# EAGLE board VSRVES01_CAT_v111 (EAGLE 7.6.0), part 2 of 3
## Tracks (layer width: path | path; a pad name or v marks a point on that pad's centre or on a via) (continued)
D4  (via drill 0.2) (continued)
  Top 0.11: TP_D8.TP 26.8,25.2 arc90 26.9,25.1 26.91,25.1 arc-90 27.01,25 27.01,25 arc-90 26.91,24.89 26.69,24.89 arc90 26.59,24.8 26.59,24.79 arc90 26.69,24.69 26.91,24.69 arc-90 27.01,24.59 27.01,24.59 arc-90 26.91,24.48 26.69,24.48 arc90 26.59,24.39 26.59,24.38 arc90 26.69,24.28 26.91,24.28 arc-90 27.01,24.18 27.01,24.18 arc-90 26.91,24.07 26.69,24.07 arc90 26.59,23.98 26.59,23.97 arc90 26.69,23.87 26.91,23.87 arc-90 27.01,23.77 27.01,23.77 arc-90 26.91,23.67 26.69,23.67 arc90 26.59,23.57 26.59,23.56 arc90 26.69,23.46 26.91,23.46 arc-90 27.01,23.36 27.01,23.36 arc-90 26.91,23.26 26.69,23.26 arc90 26.59,23.16 26.59,23.15 arc90 26.69,23.05 26.91,23.05 arc-90 27.01,22.95 27.01,22.95 arc-90 26.91,22.85 26.69,22.85 arc90 26.59,22.75 26.59,22.74 arc90 26.69,22.64 26.91,22.64 arc-90 27.01,22.54 27.01,22.54 arc-90 26.91,22.44 26.69,22.44 arc90 26.59,22.34 26.59,22.33 arc90 26.69,22.23 26.91,22.23 arc-90 27.01,22.13 27.01,22.13 arc-90 26.91,22.03 26.69,22.03 arc90 26.59,21.93 26.59,21.92 arc90 26.69,21.82 26.91,21.82 arc-90 27.01,21.72 27.01,21.72 arc-90 26.91,21.62 26.69,21.62 arc90 26.59,21.52 26.59,21.51 arc90 26.69,21.41 26.91,21.41 arc-90 27.01,21.31 27.01,21.31 arc-90 26.91,21.21 26.69,21.21 arc90 26.59,21.11 26.59,21.1 arc90 26.69,21 26.91,21 arc-90 27.01,20.9 27.01,20.9 arc-90 26.91,20.8 26.69,20.8 arc90 26.59,20.7 26.59,20.69 arc90 26.69,20.59 26.91,20.59 arc-90 27.01,20.49 27.01,20.49 arc-90 26.91,20.39 26.69,20.39 arc90 26.59,20.29 26.59,20.28 arc90 26.69,20.18 26.91,20.18 arc-90 27.01,20.08 27.01,20.08 arc-90 26.91,19.98 26.69,19.98 arc90 26.59,19.88 26.59,19.87 arc90 26.69,19.77 26.91,19.77 arc-90 27.01,19.67 27.01,19.67 arc-90 26.91,19.57 26.69,19.57 arc90 26.59,19.47 26.59,19.46 arc90 26.69,19.36 26.91,19.36 arc-90 27.01,19.26 27.01,19.26 arc-90 26.91,19.16 26.69,19.16 arc90 26.59,19.06 26.59,19.05 arc90 26.69,18.95 26.91,18.95 arc-90 27.01,18.85 27.01,18.85 arc-90 26.91,18.75 26.69,18.75 arc90 26.59,18.65 26.59,18.64 arc90 26.69,18.54 26.91,18.54 arc-90 27.01,18.44 27.01,18.44 arc-90 26.91,18.34 26.69,18.34 arc90 26.59,18.24 26.59,18.23 arc90 26.69,18.13 26.91,18.13 arc-90 27.01,18.03 27.01,18.03 arc-90 26.91,17.93 26.69,17.93 arc90 26.59,17.83 26.59,17.82 arc90 26.69,17.72 26.91,17.72 arc-90 27.01,17.62 27.01,17.62 arc-90 26.91,17.52 26.69,17.52 arc90 26.59,17.42 26.59,17.41 arc90 26.69,17.31 26.91,17.31 arc-90 27.01,17.21 27.01,17.21 arc-90 26.91,17.11 26.69,17.11 arc90 26.59,17.01 26.59,17 arc90 26.69,16.9 26.91,16.9 arc-90 27.01,16.8 27.01,16.8 arc-90 26.91,16.7 26.9,16.7 arc90 26.8,16.6 26.8,15.88 arc-90 v24.93,14
  Top 0.11: TP_D8.TP 26.8,26.4 TP_D8.TP | U1.26 26.4,27.76 26.4,27.2 26.8,26.8 TP_D8.TP
  Bottom 0.11: U100.M6 23.98,13.71 arc-45 24.69,14 v24.93,14
D5  (via drill 0.2)
  Top 0.11: v23.62,13.35 25.64,15.36 | 25.64,15.36 25.71,15.43 25.76,15.48 25.76,16.92 25.9,17.06 25.9,17.31 arc-90 26.1,17.47 26.13,17.47 arc90 26.23,17.57 26.23,17.57 arc90 26.13,17.68 25.87,17.68 arc-90 25.77,17.77 25.77,17.78 arc-90 25.87,17.88 26.13,17.88 arc90 26.23,17.98 26.23,17.99 arc90 26.13,18.09 25.87,18.09 arc-90 25.77,18.19 25.77,18.19 arc-90 25.87,18.29 26.13,18.29 arc90 26.23,18.39 26.23,18.4 arc90 26.13,18.5 25.87,18.5 arc-90 25.77,18.6 25.77,18.61 arc-90 25.87,18.7 26.13,18.7 arc90 26.23,18.8 26.23,18.81 arc90 26.13,18.91 25.87,18.91 arc-90 25.77,19.01 25.77,19.02 arc-90 25.87,19.12 26.13,19.12 arc90 26.23,19.22 26.23,19.22 arc90 26.13,19.32 25.87,19.32 arc-90 25.77,19.42 25.77,19.43 arc-90 25.87,19.53 26.13,19.53 arc90 26.23,19.63 26.23,19.63 arc90 26.13,19.73 25.87,19.73 arc-90 25.77,19.83 25.77,19.84 arc-90 25.87,19.94 26.13,19.94 arc90 26.23,20.04 26.23,20.05 arc90 26.13,20.15 25.87,20.15 arc-90 25.77,20.25 25.77,20.25 arc-90 25.87,20.35 26.13,20.35 arc90 26.23,20.45 26.23,20.46 arc90 26.13,20.56 25.87,20.56 arc-90 25.77,20.66 25.77,20.66 arc-90 25.87,20.76 26.13,20.76 arc90 26.23,20.86 26.23,20.87 arc90 26.13,20.97 25.87,20.97 arc-90 25.77,21.07 25.77,21.08 arc-90 25.87,21.18 26.13,21.18 arc90 26.23,21.28 26.23,21.28 arc90 26.13,21.38 25.87,21.38 arc-90 25.77,21.48 25.77,21.49 arc-90 25.87,21.59 26.13,21.59 arc90 26.23,21.69 26.23,21.69 arc90 26.13,21.79 25.87,21.79 arc-90 25.77,21.89 25.77,21.9 arc-90 25.87,22 26.13,22 arc90 26.23,22.1 26.23,22.11 arc90 26.13,22.2 25.87,22.2 arc-90 25.77,22.3 25.77,22.31 arc-90 25.87,22.41 26.13,22.41 arc90 26.23,22.51 26.23,22.52 arc90 26.13,22.62 25.87,22.62 arc-90 25.77,22.72 25.77,22.72 arc-90 25.87,22.82 26.13,22.82 arc90 26.23,22.92 26.23,22.93 arc90 26.13,23.03 25.87,23.03 arc-90 25.77,23.13 25.77,23.14 arc-90 25.87,23.23 26.13,23.23 arc90 26.23,23.34 26.23,23.34 arc90 26.13,23.44 25.87,23.44 arc-90 25.77,23.54 25.77,23.55 arc-90 25.87,23.65 26.13,23.65 arc90 26.23,23.75 26.23,23.75 arc90 26.13,23.85 25.87,23.85 arc-90 25.77,23.95 25.77,23.96 arc-90 25.87,24.06 26.13,24.06 arc90 26.23,24.16 26.23,24.16 arc90 26.13,24.27 25.87,24.27 arc-90 25.77,24.36 25.77,24.37 arc-90 25.87,24.47 26.13,24.47 arc90 26.23,24.57 26.23,24.58 arc90 26.13,24.68 25.87,24.68 arc-90 25.77,24.78 25.77,24.78 arc-90 25.87,24.88 26.13,24.88 arc90 26.23,24.98 26.23,24.99 arc90 26.13,25.09 25.87,25.09 arc-90 25.77,25.19 25.77,25.19 arc-90 25.87,25.29 26.13,25.29 arc90 26.23,25.39 26.23,25.4 arc90 26.13,25.5 26.1,25.5 arc-90 26,25.6 26,26.4 26,27.59 U1.25
  Top 0.11: TP_D15.TP 25.81,15.19 25.64,15.36
  Bottom 0.11: U100.L7 v23.62,13.35
D6  (via drill 0.2)
  Top 0.11: U1.24 25.6,27.43 25.6,27.2 25.2,26.8 25.2,26.4 | v22.8,12.37 22.98,12.44 22.98,12.94 arc-45 23.27,13.64 24.91,15.28 25.47,15.84 25.47,16.48 25.2,16.75 25.2,17.06 arc-90 25.3,17.16 25.36,17.16 arc90 25.46,17.26 25.46,17.27 arc90 25.36,17.37 25.04,17.37 arc-90 24.94,17.47 24.94,17.48 arc-90 25.04,17.58 25.36,17.58 arc90 25.46,17.68 25.46,17.69 arc90 25.36,17.79 25.04,17.79 arc-90 24.94,17.89 24.94,17.9 arc-90 25.04,18 25.36,18 arc90 25.46,18.1 25.46,18.11 arc90 25.36,18.21 25.04,18.21 arc-90 24.94,18.31 24.94,18.32 arc-90 25.04,18.42 25.36,18.42 arc90 25.46,18.52 25.46,18.53 arc90 25.36,18.63 25.04,18.63 arc-90 24.94,18.73 24.94,18.74 arc-90 25.04,18.84 25.36,18.84 arc90 25.46,18.94 25.46,18.95 arc90 25.36,19.05 25.04,19.05 arc-90 24.94,19.15 24.94,19.16 arc-90 25.04,19.26 25.36,19.26 arc90 25.46,19.36 25.46,19.37 arc90 25.36,19.47 25.04,19.47 arc-90 24.94,19.57 24.94,19.58 arc-90 25.04,19.68 25.36,19.68 arc90 25.46,19.78 25.46,19.79 arc90 25.36,19.89 25.04,19.89 arc-90 24.94,19.99 24.94,20 arc-90 25.04,20.1 25.36,20.1 arc90 25.46,20.2 25.46,20.21 arc90 25.36,20.32 25.04,20.32 arc-90 24.94,20.41 24.94,20.43 arc-90 25.04,20.52 25.36,20.52 arc90 25.46,20.62 25.46,20.64 arc90 25.36,20.73 25.04,20.73 arc-90 24.94,20.84 24.94,20.85 arc-90 25.04,20.95 25.36,20.95 arc90 25.46,21.05 25.46,21.06 arc90 25.36,21.16 25.04,21.16 arc-90 24.94,21.26 24.94,21.27 arc-90 25.04,21.37 25.36,21.37 arc90 25.46,21.47 25.46,21.48 arc90 25.36,21.58 25.04,21.58 arc-90 24.94,21.68 24.94,21.69 arc-90 25.04,21.79 25.36,21.79 arc90 25.46,21.89 25.46,21.9 arc90 25.36,22 25.04,22 arc-90 24.94,22.1 24.94,22.11 arc-90 25.04,22.21 25.36,22.21 arc90 25.46,22.31 25.46,22.32 arc90 25.36,22.42 25.04,22.42 arc-90 24.94,22.52 24.94,22.53 arc-90 25.04,22.63 25.36,22.63 arc90 25.46,22.73 25.46,22.74 arc90 25.36,22.84 25.04,22.84 arc-90 24.94,22.94 24.94,22.95 arc-90 25.04,23.05 25.36,23.05 arc90 25.46,23.15 25.46,23.16 arc90 25.36,23.26 25.04,23.26 arc-90 24.94,23.36 24.94,23.37 arc-90 25.04,23.47 25.36,23.47 arc90 25.46,23.57 25.46,23.58 25.46,23.74 25.2,24 TP_D7.TP
  Top 0.11: TP_D7.TP 25.2,26.4 | 25.2,26.4 TP_D7.TP
  Bottom 0.11: U100.L8 v22.8,12.37
D7  (via drill 0.2)
  Top 0.11: 24.4,15.61 24.51,16.05 arc90 24.41,16.15 arc-90 24.31,16.25 24.31,16.27 arc-90 24.41,16.37 24.61,16.37 arc90 24.71,16.47 24.71,16.49 arc90 24.61,16.59 24.41,16.59 arc-90 24.31,16.69 24.31,16.7 arc-90 24.41,16.8 24.61,16.8 arc90 24.71,16.91 24.71,16.92 arc90 24.61,17.02 24.41,17.02 arc-90 24.31,17.12 24.31,17.14 arc-90 24.41,17.24 24.61,17.24 arc90 24.71,17.34 24.71,17.36 arc90 24.61,17.46 24.41,17.46 arc-90 24.31,17.56 24.31,17.58 arc-90 24.41,17.68 24.61,17.68 arc90 24.71,17.78 24.71,17.8 arc90 24.61,17.9 24.41,17.9 arc-90 24.31,18 24.31,18.01 arc-90 24.41,18.11 24.61,18.11 arc90 24.71,18.21 24.71,18.23 arc90 24.61,18.33 24.41,18.33 arc-90 24.31,18.43 24.31,18.45 arc-90 24.41,18.55 24.61,18.55 arc90 24.71,18.65 24.71,18.67 arc90 24.61,18.77 24.41,18.77 arc-90 24.31,18.87 24.31,18.89 arc-90 24.41,18.99 24.61,18.99 arc90 24.71,19.09 24.71,19.1 arc90 24.61,19.2 24.41,19.2 arc-90 24.31,19.3 24.31,19.32 arc-90 24.41,19.42 24.61,19.42 arc90 24.71,19.52 24.71,19.54 arc90 24.61,19.64 24.41,19.64 arc-90 24.31,19.74 24.31,19.76 arc-90 24.41,19.86 24.61,19.86 arc90 24.71,19.96 24.71,19.98 arc90 24.61,20.08 24.41,20.08 arc-90 24.31,20.18 24.31,20.2 arc-90 24.41,20.3 24.61,20.3 arc90 24.71,20.39 24.71,20.41 arc90 24.61,20.51 24.41,20.51 arc-90 24.31,20.61 24.31,20.63 arc-90 24.41,20.73 24.61,20.73 arc90 24.71,20.83 24.71,20.85 arc90 24.61,20.95 24.41,20.95 arc-90 24.31,21.05 24.31,21.07 arc-90 24.41,21.17 24.61,21.17 arc90 24.71,21.27 24.71,21.29 arc90 24.61,21.39 24.41,21.39 arc-90 24.31,21.49 24.31,21.5 arc-90 24.41,21.6 24.61,21.6 arc90 24.71,21.7 24.71,21.72 arc90 24.61,21.82 24.41,21.82 arc-90 24.31,21.92 24.31,21.94 arc-90 24.41,22.04 24.61,22.04 arc90 24.71,22.14 24.71,22.16 arc90 24.61,22.26 24.41,22.26 arc-90 24.31,22.36 24.31,22.38 arc-90 24.41,22.48 24.61,22.48 arc90 24.71,22.58 24.71,22.59 arc90 24.61,22.69 24.41,22.69 arc-90 24.31,22.79 24.31,22.81 arc-90 24.41,22.91 24.61,22.91 arc90 24.71,23.01 24.71,23.03 arc90 24.61,23.13 24.41,23.13 arc-90 24.31,23.23 24.31,23.25 arc-90 24.41,23.35 24.61,23.35 arc90 24.71,23.45 24.71,23.47 arc90 24.61,23.57 24.41,23.57 arc-90 24.31,23.67 24.31,23.68 arc-90 24.41,23.79 24.61,23.79 arc90 24.71,23.89 24.71,23.9 arc90 24.61,24 24.41,24 arc-90 24.31,24.1 24.31,24.12 arc-90 24.41,24.22 24.61,24.22 arc90 24.71,24.32 24.71,24.34 arc90 24.61,24.44 24.41,24.44 arc-90 24.31,24.54 24.31,24.56 arc-90 24.41,24.66 24.61,24.66 arc90 24.71,24.76 24.71,24.78 arc90 24.61,24.88 24.41,24.88 arc-90 24.31,24.98 24.31,24.99 arc-90 24.41,25.09 24.61,25.09 arc90 24.71,25.19 24.71,25.21 arc90 24.61,25.31 24.41,25.31 arc-90 24.31,25.41 24.31,25.43 arc-90 24.41,25.53 arc90 24.51,25.63 24.51,26.26 24.4,26.37 24.4,27 24.89,27.5 U1.23
  Top 0.11: 24.4,15.61 arc-45 24.11,14.91 22.79,13.59 arc103 v22.57,13.11 | TP_D14.TP 24.34,15.55 24.4,15.61
  Bottom 0.11: 23.27,11.72 U100.L9 23.23,11.8 22.8,11.8 22.4,12.2 22.4,12.6 22.4,12.88 v22.57,13.11
D8  (via drill 0.2)
  Top 0.11: v21.43,13.12 arc103 21.2,13.6 20.8,14 20.7,14.1 20.46,14.1 19.6,14.96 19.6,15.61 19.6,16 19.69,16.09 19.88,16.41 19.88,17.61 19.4,18.2 19.4,19.65 19.48,19.72 arc-90 19.57,19.82 19.79,19.82 arc90 19.89,19.92 19.89,19.94 arc90 19.79,20.04 19.57,20.04 arc-90 19.48,20.14 19.48,20.15 arc-90 19.57,20.25 19.79,20.25 arc90 19.89,20.35 19.89,20.37 arc90 19.79,20.47 19.57,20.47 arc-90 19.48,20.57 19.48,20.58 arc-90 19.57,20.68 19.79,20.68 arc90 19.89,20.78 19.89,20.8 arc90 19.79,20.89 19.57,20.89 arc-90 19.48,21 19.48,21.01 arc-90 19.57,21.11 19.79,21.11 arc90 19.89,21.21 19.89,21.22 arc90 19.79,21.32 19.57,21.32 arc-90 19.48,21.42 19.48,21.44 arc-90 19.57,21.54 19.79,21.54 arc90 19.89,21.64 19.89,21.65 arc90 19.79,21.75 19.57,21.75 arc-90 19.48,21.85 19.48,21.87 arc-90 19.57,21.97 19.79,21.97 arc90 19.89,22.07 19.89,22.08 arc90 19.79,22.18 19.57,22.18 arc-90 19.48,22.28 19.48,22.3 arc-90 19.57,22.4 19.79,22.4 arc90 19.89,22.5 19.89,22.51 arc90 19.79,22.61 19.57,22.61 arc-90 19.48,22.71 19.48,22.73 arc-90 19.57,22.82 19.79,22.82 arc90 19.89,22.93 19.89,22.94 arc90 19.79,23.04 19.57,23.04 arc-90 19.48,23.14 19.48,23.15 arc-90 19.57,23.25 19.79,23.25 arc90 19.89,23.35 19.89,23.37 arc90 19.79,23.47 19.57,23.47 arc-90 19.48,23.57 19.48,23.58 arc-90 19.57,23.68 19.79,23.68 arc90 19.89,23.78 19.89,23.8 arc90 19.79,23.9 19.57,23.9 arc-90 19.48,24 19.48,24.01 arc-90 19.57,24.11 19.79,24.11 arc90 19.89,24.21 19.89,24.23 arc90 19.79,24.33 19.57,24.33 arc-90 19.48,24.43 19.48,24.44 arc-90 19.57,24.54 19.79,24.54 arc90 19.89,24.64 19.89,24.66 arc90 19.79,24.75 19.57,24.75 arc-90 19.48,24.86 19.48,24.87 arc-90 19.57,24.97 19.79,24.97 arc90 19.89,25.07 19.89,25.08 arc90 19.79,25.18 19.57,25.18 arc-90 19.48,25.28 19.48,25.3 arc-90 19.57,25.4 19.79,25.4 arc90 19.89,25.5 19.89,25.51 arc90 19.79,25.61 19.57,25.61 arc-90 19.48,25.71 19.48,25.73 arc-90 19.57,25.83 19.79,25.83 arc90 19.89,25.93 19.89,25.94 arc90 19.79,26.04 19.57,26.04 arc-90 19.48,26.14 19.48,26.16 arc-90 19.57,26.26 19.69,26.37 19.69,26.8
  Top 0.11: U1.15 19.89,27.51 19.69,27.31 19.69,27.01 19.69,26.8 | TP_D4.TP 19.64,26.75 19.69,26.8
  Bottom 0.11: v21.43,13.12 21.43,12.97 21.6,12.8 21.6,12.4 21.6,12 21.4,11.8 21,11.8 20.77,11.8 U100.G9
D9  (via drill 0.2)
  Top 0.11: 18.55,21.39 arc90 18.65,21.3 18.95,21.3 arc-90 19.05,21.2 19.05,21.19 arc-90 18.95,21.09 18.65,21.09 arc90 18.55,20.99 18.55,20.99 arc90 18.65,20.89 18.95,20.89 arc-90 19.05,20.79 19.05,20.79 arc-90 18.95,20.69 18.65,20.69 arc90 18.55,20.59 18.55,20.59 arc90 18.65,20.49 18.95,20.49 arc-90 19.05,20.39 19.05,20.39 arc-90 18.95,20.29 18.65,20.29 arc90 18.55,20.19 18.55,20.19 arc90 18.65,20.09 18.95,20.09 arc-90 19.05,19.99 19.05,19.98 arc-90 18.95,19.89 18.65,19.89 arc90 18.55,19.79 18.55,19.78 arc90 18.65,19.68 18.95,19.68 arc-90 19.05,19.58 19.05,19.58 arc-90 18.95,19.48 18.65,19.48 arc90 18.55,19.38 18.55,19.38 arc90 18.65,19.28 18.95,19.28 arc-90 19.05,19.18 19.05,19.18 arc-90 18.95,19.08 18.65,19.08 arc90 18.55,18.98 18.55,18.98 arc90 18.65,18.88 18.95,18.88 arc-90 19.05,18.78 19.05,18.78 arc-90 18.95,18.68 18.65,18.68 arc90 18.55,18.58 18.55,18.57 arc90 18.65,18.47 18.95,18.47 arc-90 19.05,18.37 19.05,18.37 arc-90 18.95,18.27 18.65,18.27 arc90 18.55,18.17 18.55,18.17 arc90 18.65,18.07 18.95,18.07 arc-90 19.05,17.97 19.05,17.97 arc-90 18.95,17.87 18.65,17.87 arc90 18.55,17.77 18.55,17.77 arc90 18.65,17.67 18.95,17.67 arc-90 19.05,17.57 19.05,17.57 arc-90 18.95,17.47 18.65,17.47 arc90 18.55,17.37 18.55,17.36 arc90 18.65,17.27 18.95,17.27 arc-90 19.05,17.16 19.05,17.16 arc-90 18.95,17.06 18.65,17.06 arc90 18.55,16.96 18.55,16.96 arc90 18.65,16.86 18.95,16.86 arc-90 19.05,16.76 19.05,16.76 arc-90 18.95,16.66 18.65,16.66 arc90 18.55,16.56 18.55,16.56 arc90 18.65,16.46 18.7,16.46 arc-90 18.8,16.36 18.8,16 18.81,15.99 18.81,15.34 20.35,13.8 20.6,13.8 20.73,13.67 arc-45 21.02,12.96 21.02,12.43 v21.2,12.26
  Top 0.11: 18.55,21.39 18.55,21.4 | 18.55,21.8 | U1.14 19.09,27.28 arc45 18.8,26.57 18.8,25 | 18.55,21.8 18.55,24.35 18.8,24.6 18.8,25 | 18.55,21.39 18.55,21.8 | TP_D11.TP 18.81,25.01 18.8,25
  Bottom 0.11: U100.G8 v21.2,12.26
D10  (via drill 0.2)
  Top 0.11: v20.38,13.35 19.26,14.46 19.22,14.51 18.19,15.53 18.19,18.61 18,18.8 18,18.84 arc90 17.9,18.95 17.84,18.95 arc-90 17.75,19.05 17.75,19.05 arc-90 17.84,19.15 18.16,19.15 arc90 18.25,19.25 18.25,19.26 arc90 18.16,19.36 17.84,19.36 arc-90 17.75,19.46 17.75,19.46 arc-90 17.84,19.56 18.16,19.56 arc90 18.25,19.66 18.25,19.67 arc90 18.16,19.77 17.84,19.77 arc-90 17.75,19.87 17.75,19.87 arc-90 17.84,19.97 18.16,19.97 arc90 18.25,20.07 18.25,20.08 arc90 18.16,20.18 17.84,20.18 arc-90 17.75,20.28 17.75,20.29 arc-90 17.84,20.39 18.16,20.39 arc90 18.25,20.49 18.25,20.49 arc90 18.16,20.59 17.84,20.59 arc-90 17.75,20.69 17.75,20.7 arc-90 17.84,20.8 18.16,20.8 arc90 18.25,20.9 18.25,20.9 arc90 18.16,21 17.84,21 arc-90 17.75,21.1 17.75,21.11 arc-90 17.84,21.21 18.16,21.21 arc90 18.25,21.31 18.25,21.31 arc90 18.16,21.41 17.84,21.41 arc-90 17.75,21.51 17.75,21.52 arc-90 17.84,21.62 18.16,21.62 arc90 18.25,21.72 18.25,21.73 arc90 18.16,21.83 17.84,21.83 arc-90 17.75,21.93 17.75,21.93 arc-90 17.84,22.03 18.16,22.03 arc90 18.25,22.13 18.25,22.14 arc90 18.16,22.24 17.84,22.24 arc-90 17.75,22.34 17.75,22.34 arc-90 17.84,22.44 18.16,22.44 arc90 18.25,22.54 18.25,22.55 arc90 18.16,22.65 17.84,22.65 arc-90 17.75,22.75 17.75,22.75 arc-90 17.84,22.85 18.16,22.85 arc90 18.25,22.95 18.25,22.96 arc90 18.16,23.06 17.84,23.06 arc-90 17.75,23.16 17.75,23.17 arc-90 17.84,23.27 18.16,23.27 arc90 18.25,23.37 18.25,23.37 arc90 18.16,23.47 17.84,23.47 arc-90 17.75,23.57 17.75,23.58 arc-90 17.84,23.68 18.16,23.68 arc90 18.25,23.78 18.25,23.78 arc90 18.16,23.88 17.84,23.88 arc-90 17.75,23.98 17.75,23.99 arc-90 17.84,24.09 18.16,24.09 arc90 18.25,24.19 18.25,24.19 arc90 18.16,24.29 17.84,24.29 arc-90 17.75,24.39 17.75,24.4 arc-90 17.84,24.5 17.9,24.5 arc90 18,24.6 18.29,24.89 18.29,26.8
  Top 0.11: U1.13 18.29,27.04 18.29,26.8 | TP_D3.TP 18.24,26.75 18.29,26.8
  Bottom 0.11: U100.G7 v20.38,13.35
D11  (via drill 0.2)
  Top 0.11: 17.1,19.9 17.07,19.9 | 17.07,19.9 arc-90 16.96,20 16.96,20.01 arc-90 17.07,20.11 17.34,20.11 arc90 17.43,20.21 17.43,20.22 arc90 17.34,20.32 17.07,20.32 arc-90 16.96,20.42 16.96,20.42 arc-90 17.07,20.52 17.34,20.52 arc90 17.43,20.62 17.43,20.63 arc90 17.34,20.73 17.07,20.73 arc-90 16.96,20.83 16.96,20.84 arc-90 17.07,20.94 17.34,20.94 arc90 17.43,21.04 17.43,21.05 arc90 17.34,21.15 17.07,21.15 arc-90 16.96,21.25 16.96,21.25 arc-90 17.07,21.35 17.34,21.35 arc90 17.43,21.45 17.43,21.46 arc90 17.34,21.56 17.07,21.56 arc-90 16.96,21.66 16.96,21.67 arc-90 17.07,21.77 17.34,21.77 arc90 17.43,21.87 17.43,21.88 arc90 17.34,21.98 17.07,21.98 arc-90 16.96,22.07 16.96,22.08 arc-90 17.07,22.18 17.34,22.18 arc90 17.43,22.28 17.43,22.29 arc90 17.34,22.39 17.07,22.39 arc-90 16.96,22.49 16.96,22.5 arc-90 17.07,22.6 17.34,22.6 arc90 17.43,22.7 17.43,22.7 arc90 17.34,22.8 17.07,22.8 arc-90 16.96,22.91 16.96,22.91 arc-90 17.07,23.01 17.34,23.01 arc90 17.43,23.11 17.43,23.12 arc90 17.34,23.22 17.07,23.22 arc-90 16.96,23.32 16.96,23.33 arc-90 17.07,23.43 17.34,23.43 arc90 17.43,23.53 17.43,23.53 arc90 17.34,23.63 17.07,23.63 arc-90 16.96,23.73 16.96,23.74 arc-90 17.07,23.84 17.34,23.84 arc90 17.43,23.94 17.43,23.95 arc90 17.34,24.05 17.07,24.05 arc-90 16.96,24.15 16.96,24.16 arc-90 17.07,24.26 17.34,24.26 arc90 17.43,24.36 17.43,24.36 arc90 17.34,24.46 17.07,24.46 arc-90 16.96,24.56 16.96,24.57 arc-90 17.07,24.67 17.34,24.67 arc90 17.43,24.77 17.43,24.78 arc90 17.34,24.88 17.07,24.88 arc-90 16.96,24.98 16.96,24.98 arc-90 17.07,25.09 17.34,25.09 17.34,25.09 arc90 17.43,25.19 17.43,25.19 arc90 17.34,25.29 17.07,25.29 arc-90 16.96,25.39 16.96,25.4 arc-90 17.07,25.5 17.34,25.5 arc90 17.43,25.6 17.43,25.61 arc90 17.34,25.71 17.07,25.71 arc-90 16.96,25.81 16.96,25.82 arc-90 17.07,25.91 17.2,26.05 17.2,26.4 17.2,26.52 U1.12
  Top 0.11: 17.07,19.9 17.2,19.77 17.2,19.2 17.8,18.6 17.8,15.4 19.07,14.12 v19.07,14
  Top 0.2: TP_D6.TP 17.4,26.39 17.4,26.4 17.2,26.4
  Bottom 0.11: U100.F6 20.02,13.71 arc45 19.31,14 v19.07,14
D12  (via drill 0.2)
  Top 0.11: v20.38,12.05 20.38,12.38 20.38,12.62 19.8,13.2 19.4,13.2 19.2,13 19,13 17.95,13 17.75,13.2 17.6,13.35 17.4,13.35 | U1.11 16.69,26.58 arc45 16.4,25.87 16.4,24.2 16.4,23.56 16.4,23.36 16.51,23.25 arc-90 16.61,23.15 16.61,23.13 arc-90 16.51,23.03 16.29,23.03 arc90 16.19,22.93 16.19,22.91 arc90 16.29,22.81 16.51,22.81 arc-90 16.61,22.71 16.61,22.7 arc-90 16.51,22.6 16.29,22.6 arc90 16.19,22.5 16.19,22.48 arc90 16.29,22.38 16.51,22.38 arc-90 16.61,22.28 16.61,22.26 arc-90 16.51,22.16 16.29,22.16 arc90 16.19,22.06 16.19,22.04 arc90 16.29,21.94 16.51,21.94 arc-90 16.61,21.84 16.61,21.83 arc-90 16.51,21.73 16.29,21.73 arc90 16.19,21.63 16.19,21.61 arc90 16.29,21.51 16.51,21.51 arc-90 16.61,21.41 16.61,21.39 arc-90 16.51,21.29 16.29,21.29 arc90 16.19,21.19 16.19,21.17 arc90 16.29,21.07 16.51,21.07 arc-90 16.61,20.97 16.61,20.96 arc-90 16.51,20.86 16.29,20.86 arc90 16.19,20.76 16.19,20.74 arc90 16.29,20.64 16.51,20.64 arc-90 16.61,20.54 16.61,20.52 arc-90 16.51,20.42 16.29,20.42 arc90 16.19,20.32 16.19,20.3 arc90 16.29,20.2 16.51,20.2 arc-90 16.61,20.1 16.61,20.09 arc-90 16.51,19.99 16.29,19.99 arc90 16.19,19.89 16.19,19.87 arc90 16.29,19.77 16.51,19.77 arc-90 16.61,19.67 16.61,19.65 arc-90 16.51,19.55 16.29,19.55 arc90 16.19,19.45 16.19,19.43 arc90 16.29,19.33 16.3,19.33 arc-90 16.4,19.23 16.4,19 16,18.6 16,14.6 | 17.4,13.35 17.05,13.35 arc-90 16,14.4 | 16,14.4 16,14.6 | 16,14.4 16,14.6 | TP_D16.TP 17.45,13.4 17.4,13.35
  Bottom 0.11: U100.F9 v20.38,12.05
D13  (via drill 0.2)
  Top 0.11: 15.6,25.63 arc-45 15.89,26.34 U1.10 | 15.6,25.63 15.6,25.2 arc-90 15.5,25.1 15.42,25.1 arc90 15.32,25 15.32,24.99 arc90 15.42,24.89 15.78,24.89 arc-90 15.88,24.79 15.88,24.78 arc-90 15.78,24.68 15.42,24.68 arc90 15.32,24.58 15.32,24.57 arc90 15.42,24.47 15.78,24.47 arc-90 15.88,24.37 15.88,24.36 arc-90 15.78,24.26 15.42,24.26 arc90 15.32,24.16 15.32,24.15 arc90 15.42,24.05 15.78,24.05 arc-90 15.88,23.95 15.88,23.94 arc-90 15.78,23.84 15.42,23.84 arc90 15.32,23.74 15.32,23.73 arc90 15.42,23.63 15.78,23.63 arc-90 15.88,23.53 15.88,23.52 arc-90 15.78,23.42 15.42,23.42 arc90 15.32,23.32 15.32,23.31 arc90 15.42,23.21 15.78,23.21 arc-90 15.88,23.11 15.88,23.09 arc-90 15.78,23 15.42,23 arc90 15.32,22.89 15.32,22.89 arc90 15.42,22.79 15.78,22.79 arc-90 15.88,22.68 15.88,22.67 arc-90 15.78,22.57 15.42,22.57 arc90 15.32,22.47 15.32,22.46 arc90 15.42,22.36 15.78,22.36 arc-90 15.88,22.26 15.88,22.25 arc-90 15.78,22.15 15.42,22.15 arc90 15.32,22.05 15.32,22.04 arc90 15.42,21.94 15.5,21.94 arc-90 15.6,21.84 15.6,14.8 arc90 17.7,12.7 v19.73,12.7 | TP_D10.TP 15.6,25.63
  Bottom 0.11: U100.F7 v19.73,12.7
D14  (via drill 0.2)
  Top 0.11: v19.73,12.05 17.55,12.05 arc-90 14.8,14.8 arc-90 14.97,14.97 15,14.97 arc90 15.18,15.15 15.18,15.69 arc90 15,15.87 14.6,15.87 arc-90 14.42,16.04 14.42,16.59 arc-90 14.6,16.76 15,16.76 arc90 15.18,16.93 15.18,17.48 arc90 15,17.65 14.6,17.65 arc-90 14.42,17.83 14.42,18.37 arc-90 14.6,18.55 15,18.55 arc90 15.18,18.72 15.18,19.26 arc90 15,19.44 14.6,19.44 arc-90 14.42,19.61 14.42,20.16 arc-90 14.6,20.33 15,20.33 arc90 15.18,20.51 15.18,21.05 arc90 15,21.22 14.97,21.22 arc-90 14.8,21.4 14.8,28 15.09,28.29 17.33,30.55 17.4,30.55 | U1.8 18.95,30.55 17.4,30.55 | TP_D1.TP 17.53,30.42 17.4,30.55
  Bottom 0.11: U100.F8 v19.73,12.05
D15  (via drill 0.2)
  Top 0.11: 13.76,24.56 arc90 13.86,24.46 14.14,24.46 arc-90 14.24,24.36 14.24,24.34 arc-90 14.14,24.24 13.86,24.24 arc90 13.76,24.14 13.76,24.13 arc90 13.86,24.03 14.14,24.03 arc-90 14.24,23.93 14.24,23.91 arc-90 14.14,23.81 13.86,23.81 arc90 13.76,23.71 13.76,23.7 arc90 13.86,23.6 14.14,23.6 arc-90 14.24,23.5 14.24,23.48 arc-90 14.14,23.38 13.86,23.38 arc90 13.76,23.28 13.76,23.27 arc90 13.86,23.17 13.9,23.17 arc-90 14,23.07 14,14.8 arc90 17.4,11.4 v19.07,11.4 | 13.76,24.56 13.76,24.57 | U1.7 18.65,30.8 17.2,30.8 14,27.6 14,27.4 | 14,27.4 14,25.73 14,24.8 13.76,24.56 | TP_D2.TP 14,27.4
  Bottom 0.11: U100.E8 19.37,12.34 arc45 19.07,11.64 v19.07,11.4
DA_LEFT
  Top 0.2: U7.5 2.8,20.62 2.8,22.4 3.6,23.2 7.8,23.2 9.8,25.2 9.8,35 R36.2
DA_LEFT_BUF
  Top 0.2: C47.1 0.8,43.67 0.8,33.8 0.93,33.67 C57.1 1,31.73 R43.2
DA_RIGHT
  Top 0.2: R35.2 9.6,37 9.4,36.8 9.2,36.8 8.8,36.4 8.8,33.8 9.4,33.2 9.4,25.4 7.6,23.6 4,23.6 3.48,24.12 U7.3
DA_RIGHT_BUF
  Top 0.2: R44.2 C58.1 | C58.1 8.72,30.32 | C48.1 6.2,44.12 6.2,38.6 8,36.8 8,34 7.4,33.4 7.4,31.2 8.28,30.32 C58.1
DM0B  (via drill 0.2)
  Top 0.11: v22.32,14.78 arc8 22.4,16 22.4,16.07 arc90 22.3,16.17 22.27,16.17 arc-90 22.17,16.27 22.17,16.27 arc-90 22.27,16.37 22.53,16.37 arc90 22.63,16.47 22.63,16.48 arc90 22.53,16.58 22.27,16.58 arc-90 22.17,16.68 22.17,16.69 arc-90 22.27,16.79 22.53,16.79 arc90 22.63,16.89 22.63,16.89 arc90 22.53,17 22.27,17 arc-90 22.17,17.09 22.17,17.1 arc-90 22.27,17.2 22.53,17.2 arc90 22.63,17.3 22.63,17.31 arc90 22.53,17.41 22.27,17.41 arc-90 22.17,17.51 22.17,17.52 arc-90 22.27,17.62 22.53,17.62 arc90 22.63,17.72 22.63,17.73 arc90 22.53,17.82 22.27,17.82 arc-90 22.17,17.93 22.17,17.93 arc-90 22.27,18.03 22.53,18.03 arc90 22.63,18.13 22.63,18.14 arc90 22.53,18.24 22.27,18.24 arc-90 22.17,18.34 22.17,18.35 arc-90 22.27,18.45 22.53,18.45 arc90 22.63,18.55 22.63,18.55 arc90 22.53,18.66 22.27,18.66 arc-90 22.17,18.75 22.17,18.76 arc-90 22.27,18.86 22.53,18.86 arc90 22.63,18.96 22.63,18.97 arc90 22.53,19.07 22.27,19.07 arc-90 22.17,19.17 22.17,19.18 arc-90 22.27,19.28 22.53,19.28 arc90 22.63,19.38 22.63,19.38 arc90 22.53,19.48 22.27,19.48 arc-90 22.17,19.58 22.17,19.59 arc-90 22.27,19.69 22.53,19.69 arc90 22.63,19.79 22.63,19.8 arc90 22.53,19.9 22.27,19.9 arc-90 22.17,20 22.17,20.01 arc-90 22.27,20.11 22.53,20.11 arc90 22.63,20.21 22.63,20.21 arc90 22.53,20.31 22.27,20.31 arc-90 22.17,20.41 22.17,20.42 arc-90 22.27,20.52 22.53,20.52 arc90 22.63,20.62 22.63,20.63 arc90 22.53,20.73 22.27,20.73 arc-90 22.17,20.83 22.17,20.84 arc-90 22.27,20.94 22.53,20.94 arc90 22.63,21.04 22.63,21.04 arc90 22.53,21.14 22.27,21.14 arc-90 22.17,21.24 22.17,21.25 arc-90 22.27,21.35 22.53,21.35 arc90 22.63,21.45 22.63,21.46 arc90 22.53,21.56 22.27,21.56 arc-90 22.17,21.66 22.17,21.67 arc-90 22.27,21.77 22.53,21.77 arc90 22.63,21.87 22.63,21.87 arc90 22.53,21.97 22.27,21.97 arc-90 22.17,22.07 22.17,22.08 arc-90 22.27,22.18 22.53,22.18 arc90 22.63,22.28 22.63,22.29 arc90 22.53,22.39 22.27,22.39 arc-90 22.17,22.49 22.17,22.5 arc-90 22.27,22.6 22.53,22.6 arc90 22.63,22.7 22.63,22.7 arc90 22.53,22.8 22.27,22.8 arc-90 22.17,22.9 22.17,22.91 arc-90 22.27,23.01 22.53,23.01 arc90 22.63,23.11 22.63,23.12 arc90 22.53,23.22 22.27,23.22 arc-90 22.17,23.32 22.17,23.33 arc-90 22.27,23.43 22.53,23.43 arc90 22.63,23.53 22.63,23.53 arc90 22.53,23.63 22.27,23.63 arc-90 22.17,23.73 22.17,23.74 arc-90 22.27,23.84 22.53,23.84 arc90 22.63,23.94 22.63,23.95 arc90 22.53,24.05 22.27,24.05 arc-90 22.17,24.15 22.17,24.16 arc-90 22.27,24.25 22.53,24.25 arc90 22.63,24.36 22.63,24.36 arc90 22.53,24.46 22.27,24.46 arc-90 22.17,24.56 22.17,24.57 arc-90 22.27,24.67 22.53,24.67 arc90 22.63,24.77 22.63,24.78 arc90 22.53,24.88 22.27,24.88 arc-90 22.17,24.98 22.17,24.98 arc-90 22.27,25.09 22.53,25.09 arc90 22.63,25.18 22.63,25.19 arc90 22.53,25.29 22.27,25.29 arc-90 22.17,25.39 22.17,25.4 arc-90 22.27,25.5 22.3,25.5 arc90 22.4,25.6 22.4,26 22.4,26.2 22.8,26.6 22.8,27.59 U1.20
  Bottom 0.11: U100.K5 arc45 22.42,14.68 v22.32,14.78
DM1B  (via drill 0.2)
  Top 0.11: v21.68,14.78 arc-8 21.6,16 21.69,16.05 arc-90 21.79,16.15 21.8,16.15 arc90 21.9,16.25 21.9,16.26 arc90 21.8,16.36 21.58,16.36 arc-90 21.48,16.46 21.48,16.47 arc-90 21.58,16.57 21.8,16.57 arc90 21.9,16.67 21.9,16.67 arc90 21.8,16.77 21.58,16.77 arc-90 21.48,16.87 21.48,16.88 arc-90 21.58,16.98 21.8,16.98 arc90 21.9,17.08 21.9,17.09 arc90 21.8,17.18 21.58,17.18 arc-90 21.48,17.29 21.48,17.29 arc-90 21.58,17.39 21.8,17.39 arc90 21.9,17.49 21.9,17.5 arc90 21.8,17.6 21.58,17.6 arc-90 21.48,17.7 21.48,17.7 arc-90 21.58,17.8 21.8,17.8 arc90 21.9,17.9 21.9,17.91 arc90 21.8,18.01 21.58,18.01 arc-90 21.48,18.11 21.48,18.11 arc-90 21.58,18.21 21.8,18.21 arc90 21.9,18.32 21.9,18.32 arc90 21.8,18.42 21.58,18.42 arc-90 21.48,18.52 21.48,18.53 arc-90 21.58,18.63 21.8,18.63 arc90 21.9,18.73 21.9,18.73 arc90 21.8,18.83 21.58,18.83 arc-90 21.48,18.93 21.48,18.94 arc-90 21.58,19.04 21.8,19.04 arc90 21.9,19.14 21.9,19.14 arc90 21.8,19.25 21.58,19.25 arc-90 21.48,19.34 21.48,19.35 arc-90 21.58,19.45 21.8,19.45 arc90 21.9,19.55 21.9,19.56 arc90 21.8,19.66 21.58,19.66 arc-90 21.48,19.76 21.48,19.76 arc-90 21.58,19.86 21.8,19.86 arc90 21.9,19.96 21.9,19.97 arc90 21.8,20.07 21.58,20.07 arc-90 21.48,20.17 21.48,20.18 arc-90 21.58,20.27 21.8,20.27 arc90 21.9,20.38 21.9,20.38 arc90 21.8,20.48 21.58,20.48 arc-90 21.48,20.58 21.48,20.59 arc-90 21.58,20.69 21.8,20.69 arc90 21.9,20.79 21.9,20.79 arc90 21.8,20.89 21.58,20.89 arc-90 21.48,20.99 21.48,21 arc-90 21.58,21.1 21.8,21.1 arc90 21.9,21.2 21.9,21.2 arc90 21.8,21.3 21.58,21.3 arc-90 21.48,21.41 21.48,21.41 arc-90 21.58,21.51 21.8,21.51 arc90 21.9,21.61 21.9,21.62 arc90 21.8,21.72 21.58,21.72 arc-90 21.48,21.82 21.48,21.82 arc-90 21.58,21.92 21.8,21.92 arc90 21.9,22.02 21.9,22.03 arc90 21.8,22.13 21.58,22.13 arc-90 21.48,22.23 21.48,22.23 arc-90 21.58,22.34 21.8,22.34 arc90 21.9,22.43 21.9,22.44 arc90 21.8,22.54 21.58,22.54 arc-90 21.48,22.64 21.48,22.65 arc-90 21.58,22.75 21.8,22.75 arc90 21.9,22.85 21.9,22.85 arc90 21.8,22.95 21.58,22.95 arc-90 21.48,23.05 21.48,23.06 arc-90 21.58,23.16 21.8,23.16 arc90 21.9,23.26 21.9,23.27 arc90 21.8,23.37 21.58,23.37 arc-90 21.48,23.47 21.48,23.47 arc-90 21.58,23.57 21.8,23.57 arc90 21.9,23.67 21.9,23.68 arc90 21.8,23.78 21.58,23.78 arc-90 21.48,23.88 21.48,23.88 arc-90 21.58,23.98 21.8,23.98 arc90 21.9,24.08 21.9,24.09 arc90 21.8,24.19 21.58,24.19 arc-90 21.48,24.29 21.48,24.3 arc-90 21.58,24.4 21.8,24.4 arc90 21.9,24.5 21.9,24.5 arc90 21.8,24.6 21.58,24.6 arc-90 21.48,24.7 21.48,24.71 arc-90 21.58,24.81 21.8,24.81 arc90 21.9,24.91 21.9,24.91 arc90 21.8,25.01 21.58,25.01 arc-90 21.48,25.11 21.48,25.12 arc-90 21.58,25.22 21.8,25.22 arc90 21.9,25.32 21.9,25.33 arc90 21.8,25.43 21.58,25.43 arc-90 21.48,25.53 21.48,25.53 arc-90 21.58,25.63 21.8,25.63 arc90 21.9,25.73 21.9,25.74 arc90 21.8,25.84 21.58,25.84 arc-90 21.48,25.94 21.48,25.94 arc-90 21.58,26.04 21.8,26.04 arc90 21.9,26.14 21.9,26.15 arc90 21.8,26.25 21.79,26.25 arc-90 21.69,26.35 21.6,27.11 arc-45 21.89,27.82 U1.18
  Bottom 0.11: U100.H5 arc-45 21.58,14.68 v21.68,14.78
DQSC0  (via drill 0.2)
  Top 0.11: U1.21 23.2,27.43 23.2,27.2 23.2,26.2 23.12,26.12 23.12,25.98 23.12,25.18 arc-90 23.02,25.08 22.97,25.08 arc90 22.87,24.98 22.87,24.97 arc90 22.97,24.87 23.27,24.87 arc-90 23.37,24.77 23.37,24.76 arc-90 23.27,24.66 22.97,24.66 arc90 22.87,24.56 22.87,24.56 arc90 22.97,24.46 23.27,24.46 arc-90 23.37,24.36 23.37,24.35 arc-90 23.27,24.25 22.97,24.25 arc90 22.87,24.15 22.87,24.14 arc90 22.97,24.04 23.27,24.04 arc-90 23.37,23.94 23.37,23.93 arc-90 23.27,23.83 22.97,23.83 arc90 22.87,23.73 22.87,23.72 arc90 22.97,23.62 23.27,23.62 arc-90 23.37,23.52 23.37,23.52 arc-90 23.27,23.42 22.97,23.42 arc90 22.87,23.32 22.87,23.31 arc90 22.97,23.21 23.27,23.21 arc-90 23.37,23.11 23.37,23.1 arc-90 23.27,23 22.97,23 arc90 22.87,22.9 22.87,22.89 arc90 22.97,22.79 23.27,22.79 arc-90 23.37,22.69 23.37,22.68 arc-90 23.27,22.58 22.97,22.58 arc90 22.87,22.48 22.87,22.48 arc90 22.97,22.38 23.27,22.38 arc-90 23.37,22.28 23.37,22.27 arc-90 23.27,22.17 22.97,22.17 arc90 22.87,22.07 22.87,22.06 arc90 22.97,21.96 23.27,21.96 arc-90 23.37,21.86 23.37,21.85 arc-90 23.27,21.75 22.97,21.75 arc90 22.87,21.65 22.87,21.64 arc90 22.97,21.55 23.27,21.55 arc-90 23.37,21.45 23.37,21.44 arc-90 23.27,21.34 22.97,21.34 arc90 22.87,21.24 22.87,21.23 arc90 22.97,21.13 23.27,21.13 arc-90 23.37,21.03 23.37,21.02 arc-90 23.27,20.92 22.97,20.92 arc90 22.87,20.82 22.87,20.81 arc90 22.97,20.71 23.27,20.71 arc-90 23.37,20.61 23.37,20.61 arc-90 23.27,20.5 22.97,20.5 arc90 22.87,20.41 22.87,20.4 arc90 22.97,20.3 23.27,20.3 arc-90 23.37,20.2 23.37,20.19 arc-90 23.27,20.09 22.97,20.09 arc90 22.87,19.99 22.87,19.98 arc90 22.97,19.88 23.27,19.88 arc-90 23.37,19.78 23.37,19.77 arc-90 23.27,19.67 22.97,19.67 arc90 22.87,19.57 22.87,19.57 arc90 22.97,19.46 23.27,19.46 arc-90 23.37,19.36 23.37,19.36 arc-90 23.27,19.26 22.97,19.26 arc90 22.87,19.16 22.87,19.15 arc90 22.97,19.05 23.27,19.05 arc-90 23.37,18.95 23.37,18.94 arc-90 23.27,18.84 22.97,18.84 arc90 22.87,18.74 22.87,18.73 arc90 22.97,18.63 23.27,18.63 arc-90 23.37,18.53 23.37,18.52 arc-90 23.27,18.43 22.97,18.43 arc90 22.87,18.32 22.87,18.32 arc90 22.97,18.22 23.27,18.22 arc-90 23.37,18.12 23.37,18.11 arc-90 23.27,18.01 22.97,18.01 arc90 22.87,17.91 22.87,17.9 arc90 22.97,17.8 23.27,17.8 arc-90 23.37,17.7 23.37,17.69 arc-90 23.27,17.59 22.97,17.59 arc90 22.87,17.49 22.87,17.48 arc90 22.97,17.39 23.27,17.39 arc-90 23.37,17.29 23.37,17.28 arc-90 23.27,17.18 22.97,17.18 arc90 22.87,17.08 22.87,17.07 arc90 22.97,16.97 23.27,16.97 arc-90 23.37,16.87 23.37,16.86 arc-90 23.27,16.76 22.97,16.76 arc90 22.87,16.66 22.87,16.65 arc90 22.97,16.55 23.02,16.55 arc-90 23.12,16.45 23.12,16.38 arc-25 v22.98,14.78 23.02,14.82 23.02,15.55 23.09,15.62 23.14,15.62 23.12,15.6 TP_DQSC2.TP
  Bottom 0.11: U100.L5 arc45 23.07,14.68 v22.98,14.78
DQSC1  (via drill 0.2)
  Top 0.11: U1.17 21,27.49 21,27.4 | 21,27.4 21,26.8 arc-90 20.9,26.7 20.9,26.7 arc90 20.8,26.6 20.8,26.58 arc90 20.9,26.48 21.1,26.48 arc-90 21.2,26.38 21.2,26.37 arc-90 21.1,26.27 20.9,26.27 arc90 20.8,26.17 20.8,26.15 arc90 20.9,26.05 21.1,26.05 arc-90 21.2,25.95 21.2,25.94 arc-90 21.1,25.84 20.9,25.84 arc90 20.8,25.74 20.8,25.72 arc90 20.9,25.62 21.1,25.62 arc-90 21.2,25.52 21.2,25.5 arc-90 21.1,25.4 20.9,25.4 arc90 20.8,25.3 20.8,25.29 arc90 20.9,25.19 21.1,25.19 arc-90 21.2,25.09 21.2,25.07 arc-90 21.1,24.97 20.9,24.97 arc90 20.8,24.87 20.8,24.86 arc90 20.9,24.76 21.1,24.76 arc-90 21.2,24.66 21.2,24.64 arc-90 21.1,24.54 20.9,24.54 arc90 20.8,24.44 20.8,24.42 arc90 20.9,24.32 21.1,24.32 arc-90 21.2,24.22 21.2,24.21 arc-90 21.1,24.11 20.9,24.11 arc90 20.8,24.01 20.8,23.99 arc90 20.9,23.89 21.1,23.89 arc-90 21.2,23.79 21.2,23.77 arc-90 21.1,23.68 20.9,23.68 arc90 20.8,23.57 20.8,23.56 arc90 20.9,23.46 21.1,23.46 arc-90 21.2,23.36 21.2,23.34 arc-90 21.1,23.24 20.9,23.24 arc90 20.8,23.14 20.8,23.13 arc90 20.9,23.03 21.1,23.03 arc-90 21.2,22.93 21.2,22.91 arc-90 21.1,22.81 20.9,22.81 arc90 20.8,22.71 20.8,22.7 arc90 20.9,22.59 21.1,22.59 arc-90 21.2,22.5 21.2,22.48 arc-90 21.1,22.38 20.9,22.38 arc90 20.8,22.28 20.8,22.26 arc90 20.9,22.16 21.1,22.16 arc-90 21.2,22.06 21.2,22.05 arc-90 21.1,21.95 20.9,21.95 arc90 20.8,21.85 20.8,21.83 arc90 20.9,21.73 21.1,21.73 arc-90 21.2,21.63 21.2,21.61 arc-90 21.1,21.52 20.9,21.52 arc90 20.8,21.41 20.8,21.4 arc90 20.9,21.3 21.1,21.3 arc-90 21.2,21.2 21.2,21.18 arc-90 21.1,21.08 20.9,21.08 arc90 20.8,20.98 20.8,20.97 arc90 20.9,20.87 21.1,20.87 arc-90 21.2,20.77 21.2,20.75 arc-90 21.1,20.65 20.9,20.65 arc90 20.8,20.55 20.8,20.54 arc90 20.9,20.43 21.1,20.43 arc-90 21.2,20.34 21.2,20.32 arc-90 21.1,20.22 20.9,20.22 arc90 20.8,20.12 20.8,20.1 arc90 20.9,20 21.1,20 arc-90 21.2,19.9 21.2,19.89 arc-90 21.1,19.79 20.9,19.79 arc90 20.8,19.69 20.8,19.67 arc90 20.9,19.57 21.1,19.57 arc-90 21.2,19.47 21.2,19.45 arc-90 21.1,19.36 20.9,19.36 arc90 20.8,19.25 20.8,19.24 arc90 20.9,19.14 21.1,19.14 arc-90 21.2,19.04 21.2,19.02 arc-90 21.1,18.92 20.9,18.92 arc90 20.8,18.82 20.8,18.81 arc90 20.9,18.71 21.1,18.71 arc-90 21.2,18.61 21.2,18.59 arc-90 21.1,18.49 20.9,18.49 arc90 20.8,18.39 20.8,18.37 arc90 20.9,18.27 21.1,18.27 arc-90 21.2,18.17 21.2,18.16 arc-90 21.1,18.06 20.9,18.06 arc90 20.8,17.96 20.8,17.94 arc90 20.9,17.84 21.1,17.84 arc-90 21.2,17.74 21.2,17.73 arc-90 21.1,17.63 20.9,17.63 arc90 20.8,17.53 20.8,17.51 arc90 20.9,17.41 21.1,17.41 arc-90 21.2,17.31 21.2,17.29 arc-90 21.1,17.19 20.9,17.19 arc90 20.8,17.09 20.8,17.08 arc90 20.9,16.98 21.1,16.98 arc-90 21.2,16.88 21.2,16.86 arc-90 21.1,16.76 20.9,16.76 arc90 20.8,16.66 20.8,16.65 arc90 20.9,16.55 21.1,16.55 arc-90 21.2,16.45 21.2,16.43 arc-90 21.1,16.33 20.9,16.33 arc90 20.8,16.23 20.8,16.21 arc90 20.9,16.11 20.9,16.11 arc-90 21,16.01 21,15.6 21.02,15.57 v21.02,14.78
  Top 0.11: TP_DQSC1.TP 20.99,27.39 21,27.4
  Bottom 0.11: U100.G5 arc-45 20.93,14.68 v21.02,14.78
DQST0  (via drill 0.2)
  Top 0.11: v23.62,14.97 23.62,15.22 23.62,15.62 23.8,15.8 23.8,16.04 arc90 23.7,16.14 23.68,16.14 arc-90 23.57,16.24 23.57,16.25 arc-90 23.68,16.35 23.93,16.35 arc90 24.02,16.45 24.02,16.46 arc90 23.93,16.56 23.68,16.56 arc-90 23.57,16.66 23.57,16.66 arc-90 23.68,16.76 23.93,16.76 arc90 24.02,16.86 24.02,16.87 arc90 23.93,16.97 23.68,16.97 arc-90 23.57,17.07 23.57,17.08 arc-90 23.68,17.18 23.93,17.18 arc90 24.02,17.28 24.02,17.29 arc90 23.93,17.39 23.68,17.39 arc-90 23.57,17.49 23.57,17.5 arc-90 23.68,17.6 23.93,17.6 arc90 24.02,17.7 24.02,17.7 arc90 23.93,17.8 23.68,17.8 arc-90 23.57,17.9 23.57,17.91 arc-90 23.68,18.01 23.93,18.01 arc90 24.02,18.11 24.02,18.12 arc90 23.93,18.22 23.68,18.22 arc-90 23.57,18.32 23.57,18.33 arc-90 23.68,18.43 23.93,18.43 arc90 24.02,18.53 24.02,18.54 arc90 23.93,18.64 23.68,18.64 arc-90 23.57,18.74 23.57,18.74 arc-90 23.68,18.84 23.93,18.84 arc90 24.02,18.94 24.02,18.95 arc90 23.93,19.05 23.68,19.05 arc-90 23.57,19.15 23.57,19.16 arc-90 23.68,19.26 23.93,19.26 arc90 24.02,19.36 24.02,19.37 arc90 23.93,19.47 23.68,19.47 arc-90 23.57,19.57 23.57,19.58 arc-90 23.68,19.68 23.93,19.68 arc90 24.02,19.78 24.02,19.78 arc90 23.93,19.88 23.68,19.88 arc-90 23.57,19.98 23.57,19.99 arc-90 23.68,20.09 23.93,20.09 arc90 24.02,20.19 24.02,20.2 arc90 23.93,20.3 23.68,20.3 arc-90 23.57,20.4 23.57,20.41 arc-90 23.68,20.51 23.93,20.51 arc90 24.02,20.61 24.02,20.62 arc90 23.93,20.72 23.68,20.72 arc-90 23.57,20.82 23.57,20.82 arc-90 23.68,20.92 23.93,20.92 arc90 24.02,21.02 24.02,21.03 arc90 23.93,21.13 23.68,21.13 arc-90 23.57,21.23 23.57,21.24 arc-90 23.68,21.34 23.93,21.34 arc90 24.02,21.44 24.02,21.45 arc90 23.93,21.55 23.68,21.55 arc-90 23.57,21.65 23.57,21.66 arc-90 23.68,21.76 23.93,21.76 arc90 24.02,21.86 24.02,21.86 arc90 23.93,21.96 23.68,21.96 arc-90 23.57,22.06 23.57,22.07 arc-90 23.68,22.17 23.93,22.17 arc90 24.02,22.27 24.02,22.28 arc90 23.93,22.38 23.68,22.38 arc-90 23.57,22.48 23.57,22.49 arc-90 23.68,22.59 23.93,22.59 arc90 24.02,22.69 24.02,22.7 arc90 23.93,22.8 23.68,22.8 arc-90 23.57,22.9 23.57,22.9 arc-90 23.68,23 23.93,23 arc90 24.02,23.1 24.02,23.11 arc90 23.93,23.21 23.68,23.21 arc-90 23.57,23.31 23.57,23.32 arc-90 23.68,23.42 23.93,23.42 arc90 24.02,23.52 24.02,23.53 arc90 23.93,23.63 23.68,23.63 arc-90 23.57,23.73 23.57,23.74 arc-90 23.68,23.84 23.93,23.84 arc90 24.02,23.94 24.02,23.94 arc90 23.93,24.04 23.68,24.04 arc-90 23.57,24.14 23.57,24.15 arc-90 23.68,24.25 23.93,24.25 arc90 24.02,24.35 24.02,24.36 arc90 23.93,24.46 23.68,24.46 arc-90 23.57,24.56 23.57,24.57 arc-90 23.68,24.67 23.93,24.67 arc90 24.02,24.77 24.02,24.78 arc90 23.93,24.88 23.68,24.88 arc-90 23.57,24.98 23.57,24.98 arc-90 23.68,25.08 23.93,25.08 arc90 24.02,25.18 24.02,25.19 arc90 23.93,25.29 23.68,25.29 arc-90 23.57,25.39 23.57,25.4 arc-90 23.68,25.5 23.7,25.5 arc90 23.8,25.6 23.8,25.8 23.8,25.89 23.7,25.99 23.7,26.2
  Top 0.11: U1.22 23.7,27.36 23.7,26.96 23.7,26.2 | TP_DQST1.TP 23.8,26.3 23.7,26.2
  Bottom 0.11: U100.L6 23.33,13.71 arc45 23.62,14.41 v23.62,14.97
DQST1  (via drill 0.2)
  Top 0.11: 20.4,16 20.4,16.75 arc-90 20.5,16.85 20.5,16.85 arc90 20.61,16.95 20.61,16.96 arc90 20.5,17.06 20.3,17.06 arc-90 20.2,17.16 20.2,17.18 arc-90 20.3,17.28 20.5,17.28 arc90 20.61,17.38 20.61,17.39 arc90 20.5,17.49 20.3,17.49 arc-90 20.2,17.59 20.2,17.61 arc-90 20.3,17.71 20.5,17.71 arc90 20.61,17.81 20.61,17.82 arc90 20.5,17.92 20.3,17.92 arc-90 20.2,18.02 20.2,18.04 arc-90 20.3,18.14 20.5,18.14 arc90 20.61,18.23 20.61,18.25 arc90 20.5,18.35 20.3,18.35 arc-90 20.2,18.45 20.2,18.46 arc-90 20.3,18.56 20.5,18.56 arc90 20.61,18.66 20.61,18.68 arc90 20.5,18.78 20.3,18.78 arc-90 20.2,18.88 20.2,18.89 arc-90 20.3,18.99 20.5,18.99 arc90 20.61,19.09 20.61,19.11 arc90 20.5,19.21 20.3,19.21 arc-90 20.2,19.31 20.2,19.32 arc-90 20.3,19.42 20.5,19.42 arc90 20.61,19.52 20.61,19.54 arc90 20.5,19.64 20.3,19.64 arc-90 20.2,19.74 20.2,19.75 arc-90 20.3,19.85 20.5,19.85 arc90 20.61,19.95 20.61,19.97 arc90 20.5,20.07 20.3,20.07 arc-90 20.2,20.17 20.2,20.18 arc-90 20.3,20.28 20.5,20.28 arc90 20.61,20.38 20.61,20.39 arc90 20.5,20.5 20.3,20.5 arc-90 20.2,20.59 20.2,20.61 arc-90 20.3,20.71 20.5,20.71 arc90 20.61,20.81 20.61,20.82 arc90 20.5,20.92 20.3,20.92 arc-90 20.2,21.02 20.2,21.04 arc-90 20.3,21.14 20.5,21.14 arc90 20.61,21.24 20.61,21.25 arc90 20.5,21.35 20.3,21.35 arc-90 20.2,21.45 20.2,21.47 arc-90 20.3,21.57 20.5,21.57 arc90 20.61,21.67 20.61,21.68 arc90 20.5,21.78 20.3,21.78 arc-90 20.2,21.88 20.2,21.9 arc-90 20.3,22 20.5,22 arc90 20.61,22.1 20.61,22.11 arc90 20.5,22.21 20.3,22.21 arc-90 20.2,22.31 20.2,22.32 arc-90 20.3,22.43 20.5,22.43 arc90 20.61,22.52 20.61,22.54 arc90 20.5,22.64 20.3,22.64 arc-90 20.2,22.74 20.2,22.75 arc-90 20.3,22.85 20.5,22.85 arc90 20.61,22.95 20.61,22.97 arc90 20.5,23.07 20.3,23.07 arc-90 20.2,23.17 20.2,23.18 arc-90 20.3,23.28 20.5,23.28 arc90 20.61,23.38 20.61,23.4 arc90 20.5,23.5 20.3,23.5 arc-90 20.2,23.6 20.2,23.61 arc-90 20.3,23.71 20.5,23.71 arc90 20.61,23.81 20.61,23.83 arc90 20.5,23.93 20.3,23.93 arc-90 20.2,24.03 20.2,24.04 arc-90 20.3,24.14 20.5,24.14 arc90 20.61,24.24 20.61,24.25 arc90 20.5,24.36 20.3,24.36 arc-90 20.2,24.45 20.2,24.47 arc-90 20.3,24.57 20.5,24.57 arc90 20.61,24.67 20.61,24.68 arc90 20.5,24.78 20.3,24.78 arc-90 20.2,24.88 20.2,24.9 arc-90 20.3,25 20.5,25 arc90 20.61,25.1 20.61,25.11 arc90 20.5,25.21 20.3,25.21 arc-90 20.2,25.31 20.2,25.33 arc-90 20.3,25.43 20.5,25.43 arc90 20.61,25.53 20.61,25.54 arc90 20.5,25.64 20.3,25.64 arc-90 20.2,25.74 20.2,25.76 arc-90 20.3,25.86 20.5,25.86 arc90 20.61,25.96 20.61,25.97 arc90 20.5,26.07 20.3,26.07 arc-90 20.2,26.17 20.2,26.19 arc-90 20.3,26.29 20.5,26.29 arc90 20.61,26.39 20.61,26.4 arc90 20.5,26.5 20.5,26.5 arc-90 20.4,26.6 20.4,27.04 arc-45 20.69,27.75 U1.16
  Top 0.11: 20.4,16 arc-3 v20.38,14.78 | 20.4,16 TP_DQST2.TP
  Bottom 0.11: U100.G6 20.67,13.71 arc-45 20.38,14.41 v20.38,14.78
GND  (via drill 0.2, 0.3, 0.4)
  Top 0.11: C69.2 12.47,16.68 v12.2,16.4 | C73.2 22.48,9.53 22,9.4 v22,8.8 | R45.1 32.75,24.15 v32.8,24.2
  Top 0.2: U1.P$4 22.14,35.41 U1.79 18.6,38.95 18.6,39.8 18.2,40.2 | C67.2 32.88,17.27 v32.8,17.2 | C50.2 v28.2,44.2 | C45.2 v20.2,48 | C44.2 v18.6,48 | C76.2 v23.6,7.8 | U6.4 45.7,23.09 45.7,23 | R61.1 47.6,6.4 v48.4,6.4 | R57.1 40.65,8.45 | C43.2 41.8,49.4 | v55.4,58.2 RP2.7 RP2.5 RP2.3 RP2.1 | C35.2 C34.2 v49,52.6 49.08,52.52 C40.2 C39.2 | U2.29 48.06,62.8 U2.G6 | RP1.3 v57,69.6 | RP1.5 v57,70.4 | RP1.7 v57,71.2 | XTAL1.2 46.1,75.3 v45.2,76.2 44.3,77.1 XTAL1.4 | C11.2 v35.8,71.6 | C10.2 v34.2,71.6 | C12.2 v37.4,71.4 | C13.2 v39,71.4 | C9.2 v40,72.4 | C14.2 40.6,71.2 v40.8,71.4 | C15.2 42.2,71.4 v42,71.6 | U4.11 v7.2,40.4 | U4.3 2.35,41.05 2.4,41 v3,41 | C55.2 v2.2,33.4 | R40.1 6.65,30.95 v6.6,31.6 | C58.2 v8.4,33 | C26.2 7.6,56.8 v8,56.4 | C25.2 v3,59 | C27.2 v9.4,60.2 | U7.4 v2.2,25 | C33.2 47,53 v46.6,52.6 | C32.2 44.8,53 v44.4,52.6 | C38.2 42.67,51.12 | C37.2 42.12,51.12 | RP4.7 v56.2,49.6 | RP4.5 55.6,48.8 v56.2,48.2 56,48 RP4.3 | RESET.P2 10.12,4.8 | 10.12,4.8 RESET.P1 | v11.2,4.8 10.12,4.8 | 16.3,39.4 C52.2
  Top 0.3: R59.1 23.6,6.2 v23.8,6.4 | C74.2 v18,8 | 9.35,18.95 9.2,19 | C53.2 14.53,37.73 14.4,37.4 14.36,37.44 v13.49,37.44 | C56.2 v12.8,35 | C28.1 15.53,54.88 v15.6,54.8 | C29.1 21.27,54.92 v21.4,54.8 | v14.6,48.6 14.32,48.88 C41.1 14.32,49.67 13.4,50.6 13.4,54.8 14.4,55.8 15.6,55.8 | C42.1 22.48,49.27 v21.8,48.6 | C49.2 32.67,43.08 32.8,43.2 v33.8,43.2 | C75.2 v25,7.2 | R51.1 9.35,15.25 9.4,15.2 v9.4,14.5 | 41.8,49.4 v41.8,48.5 | R18.2 v34.8,63 | v56.4,22.3 USD.9 v58.6,22.3 | v56.6,32.8 USD.10 56.65,33.05 v56.6,34.2 | C51.2 11.8,39.33 v11.8,38.6 | R32.2 10.6,42.85 v10.6,43.4 10.6,43.92 C46.2 | U5.4 v9.8,64 | C18.2 10.6,64.88 v10.6,64.2 | R27.1 11.15,54.45 v11,54.6 | R29.1 v11.8,50.8 | 42.67,51.12 v42.4,51.1 42.12,51.12 | C17.2 39.4,67 v39,66.6 | C19.2 v56.4,67.4 | R20.1 v56,63 | C16.2 51.48,70.47 v51.9,70.5 | R6.1 51.05,73.15 v51,73.5 | C8.2 46.6,73.8 v46.8,74 | C6.2 v42.4,78 | C3.2 v43.4,78.8 | C2.2 v43.4,80.2 | C70.2 v42.2,17.8 | U8.2 v44.8,16.4 | U9.2 v50.6,16.4 | U10.2 v56.4,16.4 | 18.2,40.2 17.1,40.2 16.3,39.4
  Top 0.4: 45.7,23 v45.7,21.4 | C59.2 v39.8,24.2 | C60.2 50.6,26.4 v50.6,27.3 | 6.4,22.2 C62.2 6.4,22.3 v7.3,22.3 | X1.G3 v58.1,3.2 | v52.6,3.2 X1.G1 v50.7,3.2 | R64.1 v52.6,1.2 | C24.2 v36.2,58.8 | C30.2 36.92,55.2 v36.2,55.2 | v4.2,65.2 3.2,65.2 R11.1 3.2,65 | USD.6 56.4,25.65 56.4,25.6
  Bottom 0.1: 20.05,14.35 19.8,14.63 18.4,14.63 18.38,14.6 U100.C5 | 18.07,14.32 17.8,14.63 17,14.63 16.8,14.4
  Bottom 0.11: 18.93,22.88 v18.97,22.96 | 24.4,31 U1.P$9 | C111.2 28,31 27.6,31.4 27.6,33.47 27.6,33.63 | C101.2 v31.6,12 | C110.2 v17,29.2 | C112.2 20.65,33.08 U1.P$7 | C106.2 13.72,19.68 13.4,20 | U100.C9 U100.D10 18.75,11.05 | U100.G10 20.7,11.1 | U100.J8 22,12.2 23,11.2 23.18,11.2 U100.L10 23.32,11.07 | U100.N10 24.6,11 v25,10.6 25.25,10.85 U100.P10 U100.R9 | U100.R5 U100.R6 | U100.M5 23.95,14.35 24.4,14.8 25.43,14.8 U100.R5 | U100.R5 26.1,14.5 26.4,14.8 26.8,14.8 v27,14.6 | U100.F5 20.05,14.35 | U100.C5 18.07,14.32 | 16.8,14.4 16.8,14.37 v16.67,14.3 | U100.J5 22.07,14.32 v22.32,14.01 | U100.D1 18.75,16.73 19.06,16.41 19.06,16.04 | 19.06,16.04 19.17,15.94 19.61,15.94 19.72,16.05 | 19.72,16.05 19.72,16.41 19.48,16.65 19.48,16.84 U100.E1 | U100.C2 18.27,16.27 18.58,15.96 19,15.96 19.06,16.04 | U100.H2 21.29,16.27 20.98,15.95 19.8,15.95 19.72,16.05 | U100.N1 U100.P1 U100.R2 25.95,16.27 v26.22,16.59 | C102.2 12.93,13.07 C103.2 | U100.C6 18.12,13.68 | U100.J1 22,19.67 22.29,19.96 22.29,21.16 22.66,21.53 v29,21.53
  Bottom 0.2: C107.2 18.93,22.88 | C105.2 32.4,16.8 v32.8,17.2 | C104.2 v31.8,14 | 18.75,11.05 v19.2,10.6 19.4,10.8 U100.E10 | 20.7,11.1 v20.38,11.39 | 23.32,11.07 v23.61,11.39 | U100.E1 v19.4,17.4 | 18.12,13.68 v18.41,13.36 | 46.4,53.4 C114.2 46.4,52.8 v46.6,52.6
  Bottom 0.3: 27.6,33.63 U1.P$3 27.5,34.27 C113.2 | C100.2 12.4,10.6 v12.2,10.8 | 12.93,13.07 v13,13 | C111.2 27.6,30.68 27.6,33.47 27.49,33.58 27.49,33.79 27.29,33.99 27.26,33.99 | C119.2 42.87,62.12 U2.G1 | C118.2 U2.G6 | C108.2 25.93,28.88 24.4,30.4 | 24.4,30.4 24.4,31 24.4,31.2 | C109.2 22.88,28.88 24.4,30.4 | C112.2 20.68,33.08 21.6,34 | C121.2 39.2,66.4 v39,66.6 | 37.4,56.2 C115.2 37,56
  Bottom 0.4: 13.4,20 v13.4,20.6 | C120.2 46.2,64.4 U2.G3 | 37,56 v36.2,56 | C117.2 37.33,61.6 v36.2,61.6
  other vias: 9.4,20.2 13.2,39.4 38.8,4.8 37.6,82 37.6,78.8 35.6,61.1 7.2,68.6 48,17.8 53.8,17.8 35.8,4.8 32,4.8 58,11.6 52.6,11.6 3.8,31.8 2.1,30.2 34.2,53.6 37.6,80.4 37.8,77 4.2,64.2 56.2,25.6 53.8,25.3 49.6,33.9 52.6,35.3
  pour GND (isolate 0.4): 0,85.6 0,0 60,0 60,85.6
  pour Top (isolate 0.4, rank 2): 0,85.6 60,85.6 60,0 0,0
  pour Bottom (isolate 0.4, rank 2): 0,85.6 60,85.6 60,0 0,0
GND1
  Top 0.3: C5.1 34.92,78.88
  Top 0.4: C4.1 C1.1 C5.1 34.92,77 FB1.1 34.8,75 34.08,74.28 J1.S2 J1.S1
GP0  (via drill 0.3)
  Top 0.2: U1.61 27.2,39.91 27.2,44 29,45.8 v29.4,45.8 29.6,45.8 30.6,46.8 32.6,46.8 v33.2,47.4 | v39,34.4 39,31.8 37.6,30.4 37.6,10.55 R57.2 38.95,8.88 BUT1.S2 v37.88,3.8 BUT1.S1
  Bottom 0.2: v33.2,47.4 33.2,46.8 36.8,43.2 36.8,38.4 39,36.2 v39,34.4 | JP2.2 31,4.4 31.6,3.8 v37.88,3.8
GP1  (via drill 0.3)
  Top 0.2: U1.62 26.8,40.08 26.8,44.2 29.2,46.6 v29.4,46.6 29.6,46.6 v31.8,48.8 | v39.8,34.4 39.8,33 39.6,32.8 39.6,31.8 38,30.2 38,12 38.8,11.2 45.2,11.2 46.2,10.2 46.2,8.32 BUT2.S2 v45.67,4 BUT2.S1 46.4,1.8 47.6,3 R61.2
  Bottom 0.2: v31.8,48.8 32.6,48.8 33.8,47.6 33.8,46.8 37.4,43.2 37.4,38.6 39.8,36.2 v39.8,34.4 | JP2.1 33.06,6.94 34.2,5.8 38.8,5.8 40.6,4 v45.67,4
GP4_SPI_SCK  (via drill 0.3)
  Top 0.2: U1.65 25.6,40.57 25.6,45 30.4,49.8 32.6,49.8 v35.8,46.6 | U6.6 44.4,29.23 44.4,31.4 43.85,31.95 R66.1 42.4,32 v40.6,32
  Bottom 0.2: v35.8,46.6 41.4,41 41.4,34.6 40.6,33.8 v40.6,32 43.8,32 44.4,31.4 49.2,31.4 49.6,31.8 U11.2
GP5_SPI_XCS  (via drill 0.3)
  Top 0.2: U1.63 26.4,40.24 26.4,44.4 v29.4,47.4 | v36.6,35.4 36.6,29.8 v37,29.4 | v34.9,43.1 35.8,44 39.8,44 40.2,43.6 LE.A RE.A 43.2,43 | JP1.1 27.35,55.02 R62.1 | U6.1 39.2,23.2 38.8,23.6 38.8,28.2 39.4,28.8 v39.4,29.4
  Bottom 0.2: JP1.1 27.33,47.87 27.8,47.4 v29.4,47.4 30.6,47.4 v34.9,43.1 34.9,37.7 36.6,36 v36.6,35.4 | U11.1 50.55,31.35 50.2,31 44.4,31 43.8,30.4 41.6,30.4 40.6,29.4 v39.4,29.4 v37,29.4
GP6_SPI_MISO  (via drill 0.3)
  Top 0.2: U1.66 25.2,40.74 25.2,45.2 30.2,50.2 32.8,50.2 35.6,47.4 37,47.4 v37.4,47 | 43.2,23.23 U6.2 43.16,21.57 42.8,21.2 40.2,21.2 38.4,23 38.4,30 40,31.6 40,32.4 40.4,32.8 v41.2,32.8
  Bottom 0.2: v37.4,47 43.6,40.8 43.6,38.6 43.35,38.35 R3.1 42.2,38.35 42.2,33 42,32.8 v41.2,32.8
GP7_SPI_MOSI  (via drill 0.3)
  Top 0.2: U1.64 26,40.41 26,44.8 30.6,49.4 32.2,49.4 v34.6,47 | v40.6,34.8 43.2,34.8 43.6,34.4 43.6,33 44.4,32.2 45,32.2 45.7,31.5 U6.5
  Bottom 0.2: v34.6,47 34.6,46.6 38,43.2 38,39.4 39.05,38.35 R4.1 40.6,38.35 v40.6,34.8
GP8_SD_CLK  (via drill 0.3)
  Top 0.2: U1.69 23.21,40 23.2,40 22.8,40.4 22.8,41.2 24,42.4 24,45.8 27,48.8 27,49.4 28.2,50.6 33,50.6 35.8,47.8 37.6,47.8 v38.4,47 | v44.2,33.2 46,33.2 46.2,33 47.4,33 47.8,32.6 47.8,30.2 49.2,28.8 49.2,26 49.8,25.4 52.8,25.4 54.2,26.8 54.9,26.8 USD.5
  Bottom 0.2: v38.4,47 44.2,41.2 v44.2,33.2
GP9_SD_CMD  (via drill 0.3)
  Top 0.2: U1.70 22.4,40.24 22.4,41.4 23.6,42.6 23.6,46 26.6,49 26.6,49.6 28,51 33.2,51 36,48.2 38,48.2 v39.6,46.6 | v44.8,34 45.8,34 46.4,33.4 47.6,33.4 48.2,32.8 48.2,30.4 49.8,28.8 RP6.7 50.6,28.2 50.8,28 53,28 53.95,28.95 USD.3
  Bottom 0.2: v39.6,46.6 44.8,41.4 v44.8,34
GP10_SD_DAT0  (via drill 0.3)
  Top 0.2: U1.71 22,40.08 22,41.6 23.2,42.8 23.2,46.2 26.2,49.2 26.2,49.8 27.8,51.4 33.4,51.4 36.2,48.6 38.6,48.6 v40.2,47 | v45.4,32.6 47,32.6 47.4,32.2 v47.4,29.6 48.8,28.2 48.8,25.8 49.6,25 53,25 53.4,24.6 54.8,24.6 | RP6.5 v49.8,29.6
  Top 0.4: USD.7 54.85,24.55 54.8,24.6
  Bottom 0.2: v40.2,47 45.4,41.8 v45.4,32.6 | v47.4,29.6 v49.8,29.6
GP11_SD_DAT1  (via drill 0.3)
  Top 0.2: U1.73 21.2,39.75 21.2,42 22.4,43.2 22.4,46.6 25.4,49.6 25.4,50.2 27.4,52.2 33.8,52.2 36.6,49.4 39.4,49.4 41.6,47.2 v42.2,47.2 | v46.6,32 46.6,31.2 46.8,31 46.8,29.4 48.4,27.8 48.4,23.4 48.8,23 52,23 52.2,23.2 52.2,24 R46.1 53.2,24 53.75,23.45 USD.8
  Bottom 0.2: v42.2,47.2 46.6,42.8 v46.6,32
GP12_SD_DAT2  (via drill 0.3)
  Top 0.2: U1.72 21.6,39.91 21.6,41.8 22.8,43 22.8,46.4 25.8,49.4 25.8,50 27.6,51.8 33.6,51.8 36.4,49 39.2,49 v41.6,46.6 | v46,34.8 47.4,34.8 49,33.2 49,31.6 49.4,31.2 RP6.1 50.6,31.8 50.8,32 53,32 53.85,31.15 USD.1
  Bottom 0.2: v41.6,46.6 46,42.2 v46,34.8
GP13_SD_DAT3  (via drill 0.3)
  Top 0.2: U1.74 20.8,39.58 20.8,42.2 22,43.4 22,46.8 25,49.8 25,50.4 27.2,52.6 34,52.6 36.8,49.8 39.6,49.8 41.6,47.8 42.4,47.8 v43.6,46.6 | v47.2,34 47.6,34 48.6,33 48.6,31.2 v49.4,30.4 RP6.3 | USD.2 53.6,30.05 v53.2,30.4
  Bottom 0.2: v43.6,46.6 47.2,43 v47.2,34 | v53.2,30.4 v49.4,30.4
HP_LEFT  (via drill 0.4)
  Top 0.2: U4.2 3.3,41.7 | 6.2,47 6.4,47.2 | 10.25,48.15 v10.2,48.2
